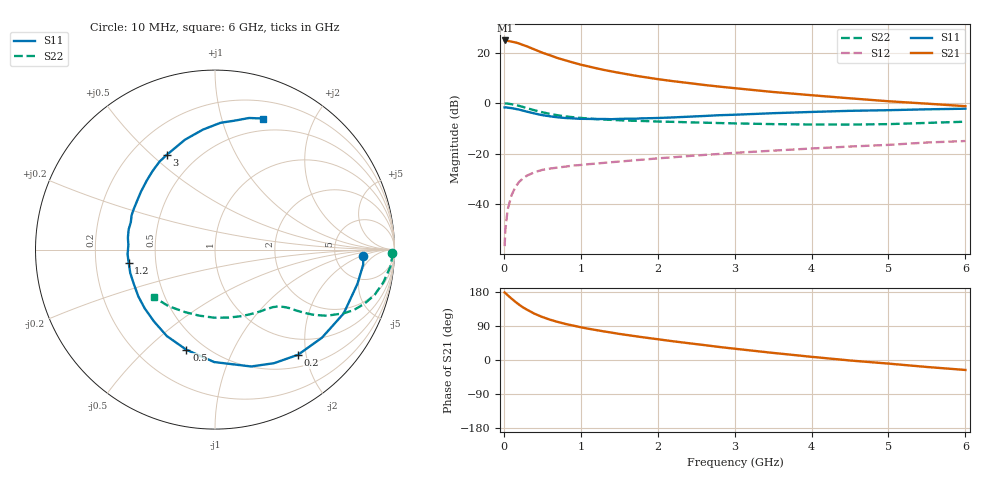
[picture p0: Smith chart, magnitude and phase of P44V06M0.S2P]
! SIEMENS Small Signal Semiconductors
! BFP182
! Si NPN RF Bipolar Junction Transistor in SOT143
! VCE = 4 V  IC = 6 mA
! Common Emitter S-Parameters:  March  1996
# GHz  S  MA  R  50
!  f  S11  S21  S12  S22
! GHz  MAG  ANG  MAG  ANG  MAG  ANG  MAG  ANG
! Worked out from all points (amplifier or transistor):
!   36 points, 10 MHz to 6 GHz, reference 50 ohm
!   highest |S21| = 24.8 dB at 20 MHz (marker M1)
!   |S21| within 3 dB of that: start of sweep to 353.9 MHz
!   unconditionally stable (mu >= 1): 1.496 GHz to 5.452 GHz
!   at 250 MHz: K = 0.23, MSG = 26.3 dB, |S12| = -29.7 dB
!   at 1.4 GHz: K = 0.97, MSG = 17.9 dB, |S12| = -23.3 dB
!   at 6 GHz: K = 0.94, MSG = 6.9 dB, |S12| = -14.9 dB
!   lowest NFmin = 1.25 dB at 450 MHz
!   S11 on the Smith chart (normalised r, x): 10 MHz: 10, -2; 200 MHz: 0.70, -1.85; 500 MHz: 0.40, -0.67; 1.2 GHz: 0.35, -0.07; 3 GHz: 0.34, +0.56; 6 GHz: 0.37, +1.37
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0.01  0.8251 -2.6  17.1 178.2  0.0015 87.9  0.9886 -1.1
0.02  0.8301 -5.7  17.36 176.7  0.0032 84.2  0.9885 -2.3
0.05  0.8161 -13.6  17.05 170.8  0.008 85.0  0.9822 -5.5
0.1  0.8003 -26.4  16.45 162.0  0.0152 75.5  0.9561 -10.9
0.15  0.772 -39.5  15.88 153.5  0.0221 69.4  0.9247 -15.8
0.2  0.7466 -51.7  15.08 145.8  0.0281 64.7  0.8857 -19.9
0.25  0.7133 -62.5  14.11 138.7  0.0328 60.0  0.8429 -23.6
0.3  0.6816 -72.8  13.28 132.9  0.0371 55.7  0.7989 -26.4
0.4  0.6266 -90.4  11.5 122.0  0.0434 49.6  0.7238 -30.6
0.5  0.5805 -105.9  9.955 113.5  0.0482 45.0  0.6636 -33.3
0.6  0.5515 -119.1  8.843 106.4  0.0512 42.0  0.6149 -35.1
0.7  0.5254 -130.2  7.782 100.5  0.0535 40.3  0.578 -36.4
0.8  0.5105 -140.1  7.032 95.2  0.0559 38.8  0.5503 -37.4
1.1  0.4899 -164.4  5.326 82.5  0.0625 36.7  0.4977 -39.9
1.2  0.4867 -171.1  4.908 79.0  0.0641 36.3  0.4866 -40.9
1.7  0.493 162.2  3.514 63.1  0.0748 36.4  0.4493 -46.2
2.2  0.5239 141.9  2.723 49.4  0.0856 35.8  0.4281 -53.3
3  0.5919 117.1  1.983 29.8  0.1046 33.4  0.3995 -68.0
3.5  0.6348 105.3  1.666 18.7  0.1156 30.7  0.3863 -78.8
4.5  0.7072 87.5  1.249 -1.3  0.1393 25.3  0.3784 -103.6
5.5  0.7574 75.5  0.98 -18.4  0.1674 19.5  0.4082 -129.5
6  0.7786 69.7  0.874 -26.3  0.1791 15.1  0.4312 -142.1
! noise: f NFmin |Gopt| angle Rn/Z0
0.45  1.25  0.25  39  0.3
0.9  1.4  0.25  78  0.23
1.8  1.95  0.21  151  0.2
